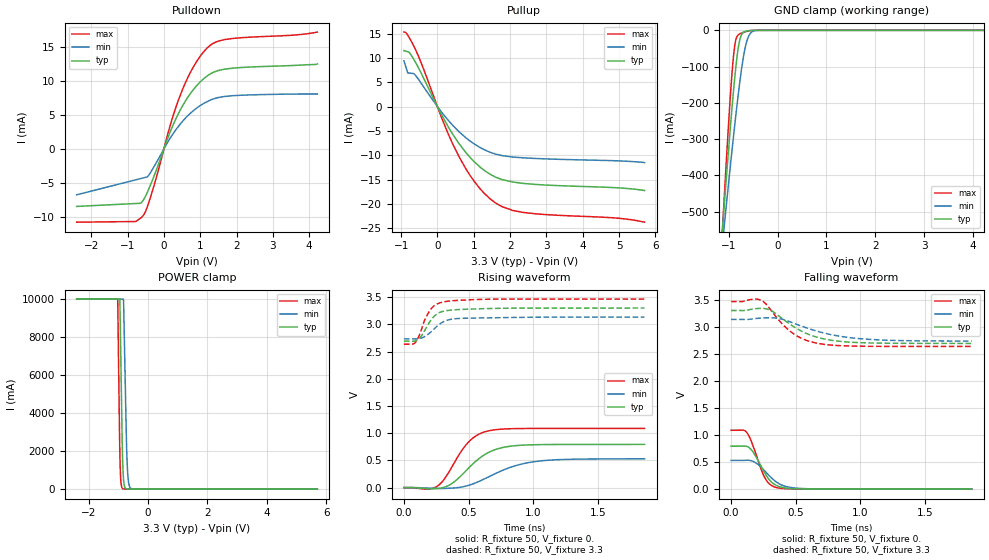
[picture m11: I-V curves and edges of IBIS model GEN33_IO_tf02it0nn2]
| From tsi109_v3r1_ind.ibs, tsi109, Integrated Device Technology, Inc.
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|   MODEL GEN33_IO_tf02it0nn2
[Model]   GEN33_IO_tf02it0nn2
Model_type  I/O
C_comp 1.184p 1.094p 1.271p
Polarity   Non-Inverting
Enable   Active-High
|   typ   min   max
Vinl   =   0.800v
Vinh   =   2.000v
Vmeas  =   1.65V
[Model Spec]
[Temperature Range]   25   125   -40
[Voltage Range] 3.3 3.135 3.465
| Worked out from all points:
|   slope of the pulldown table from 0 to 0.495 V, typ, clamps not added: 80 ohm
|   slope of the pullup table from 0 to 0.495 V, typ, clamps not added: 76.2 ohm
|   GND clamp passes 1 mA (typ) near -0.60 V on its own axis
|   POWER clamp passes 1 mA (typ) near -0.62 V on its own axis
|   rising waveform, R_fixture 50, V_fixture 0.: 20-80 % time 230ps typ, 323ps min, 184ps max; typ from 0 V to 0.794 V
|   rising waveform, R_fixture 50, V_fixture 3.3: 20-80 % time 107ps typ, 127ps min, 95.7ps max; typ from 2.69 V to 3.3 V
|   falling waveform, R_fixture 50, V_fixture 0.: 20-80 % time 118ps typ, 144ps min, 101ps max; typ from 0.794 V to 0 V
|   falling waveform, R_fixture 50, V_fixture 3.3: 20-80 % time 275ps typ, 373ps min, 221ps max; typ from 3.3 V to 2.69 V
[Pulldown]
-2.4V     -8.474mA   -6.758mA   -10.8mA
-792.5mV  -8.051mA   -4.575mA   -10.71mA
-645.1mV  -8.005mA   -4.374mA   -10.22mA
-564.7mV  -7.544mA   -4.265mA   -9.794mA
-397.3mV  -5.675mA   -3.724mA   -7.603mA
-176.3mV  -2.658mA   -1.719mA   -3.616mA
192.1mV   2.763mA    1.758mA    3.814mA
460.1mV   5.843mA    3.744mA    8.065mA
841.9mV   8.967mA    5.789mA    12.39mA
1.271V    11.07mA    7.197mA    15.29mA
1.9V      11.94mA    7.873mA    16.33mA
4.224V    12.56mA    8.123mA    17.26mA
[Pullup]
-924.4mV  11.54mA    9.439mA    15.35mA
-817.2mV  11.3mA     6.948mA    14.7mA
-656.5mV  9.808mA    6.804mA    12.54mA
-522.5mV  7.998mA    5.632mA    10.38mA
127.2mV   -1.863mA   -1.26mA    -2.522mA
596.1mV   -7.614mA   -5.158mA   -10.31mA
1.005V    -11.27mA   -7.626mA   -15.29mA
1.453V    -13.91mA   -9.382mA   -18.97mA
1.775V    -14.98mA   -10.06mA   -20.55mA
2.364V    -15.78mA   -10.51mA   -21.75mA
4.977V    -16.69mA   -11.14mA   -22.93mA
5.7V      -17.24mA   -11.51mA   -23.75mA
[GND Clamp]
-2.4V     -2.994A    -2.407A    -3.893A
-1.148V   -581.3mA   -613.7mA   -592.9mA
-1.116V   -523.7mA   -570.4mA   -515.1mA
-1.084V   -466.7mA   -527.3mA   -438.6mA
-980.4mV  -288mA     -390.1mA   -205.8mA
-908.6mV  -174.3mA   -298.6mA   -77.7mA
-852.8mV  -97.7mA    -230.6mA   -24.92mA
-781mV    -29.94mA   -149.4mA   -10.11mA
-701.2mV  -5.515mA   -73.96mA   -5.608mA
-637.4mV  -1.851mA   -32.79mA   -3.005mA
-477.9mV  -98.73uA   -1.277mA   -164.1uA
4.224V    0A         0A         0A
[Power Clamp]
-2.4V     10A        10A        10A
-1.018V   10A        10A        9.953A
-947.4mV  10A        10A        1.932A
-939.5mV  9.313A     10A        1.392A
-908mV    6.281A     10A        333.8mA
-852.7mV  1.498A     10A        28.72mA
-821.1mV  483.4mA    9.885A     10.82mA
-734.3mV  19.62mA    3.196A     4.062mA
-702.7mV  6.965mA    1.436A     3.296mA
-655.3mV  2.051mA    388.5mA    2.318mA
-584.3mV  591.6uA    50.79mA    1.148mA
5.7V      0A         0A         0A
[Ramp]
dV/dt_r .476/230.063p .318/323.059p .653/183.508p
dV/dt_f .365/274.969p .241/374.442p .498/220.766p
[Rising Waveform]
R_fixture = 50
V_fixture = 0.
0s        0V         0V         0V
175ps     -18.58mV   -7.316mV   -28.75mV
255ps     -17.18mV   -15.31mV   20.26mV
310ps     5.743mV    -15.55mV   149.1mV
375ps     81.29mV    -8.553mV   395.9mV
495ps     346.3mV    37.75mV    825.6mV
650ps     640.6mV    191.6mV    1.04V
795ps     750.9mV    347.9mV    1.079V
1.025ns   788.5mV    481.4mV    1.087V
1.86ns    793.7mV    530.4mV    1.088V
[Rising Waveform]
R_fixture = 50
V_fixture = 3.3
V_fixture_min = 3.135
V_fixture_max = 3.465
0s        2.691V     2.733V     2.636V
85ps      2.693V     2.731V     2.658V
110ps     2.725V     2.734V     2.751V
130ps     2.771V     2.745V     2.866V
160ps     2.883V     2.775V     3.072V
210ps     3.081V     2.863V     3.283V
255ps     3.189V     2.963V     3.373V
315ps     3.246V     3.058V     3.417V
505ps     3.28V      3.114V     3.451V
1.86ns    3.3V       3.135V     3.465V
[Falling Waveform]
R_fixture = 50
V_fixture = 0.
0s        793.7mV    530.7mV    1.088V
95ps      796mV      531.3mV    1.089V
120ps     790.8mV    533.9mV    1.052V
165ps     703.5mV    518.9mV    829.5mV
255ps     321.5mV    348.6mV    236.4mV
295ps     175.3mV    248.6mV    99.82mV
355ps     63.82mV    124mV      26.66mV
435ps     17.77mV    43.75mV    7.837mV
570ps     4.592mV    9.819mV    2.576mV
1.86ns    2.98uV     32.28uV    894.2nV
[Falling Waveform]
R_fixture = 50
V_fixture = 3.3
V_fixture_min = 3.135
V_fixture_max = 3.465
0s        3.3V       3.135V     3.465V
230ps     3.34V      3.16V      3.491V
310ps     3.298V     3.166V     3.3V
395ps     3.152V     3.139V     3.053V
470ps     3.023V     3.078V     2.892V
555ps     2.906V     3.002V     2.775V
670ps     2.803V     2.914V     2.693V
830ps     2.733V     2.828V     2.652V
1.05ns    2.702V     2.769V     2.639V
1.86ns    2.692V     2.734V     2.636V
